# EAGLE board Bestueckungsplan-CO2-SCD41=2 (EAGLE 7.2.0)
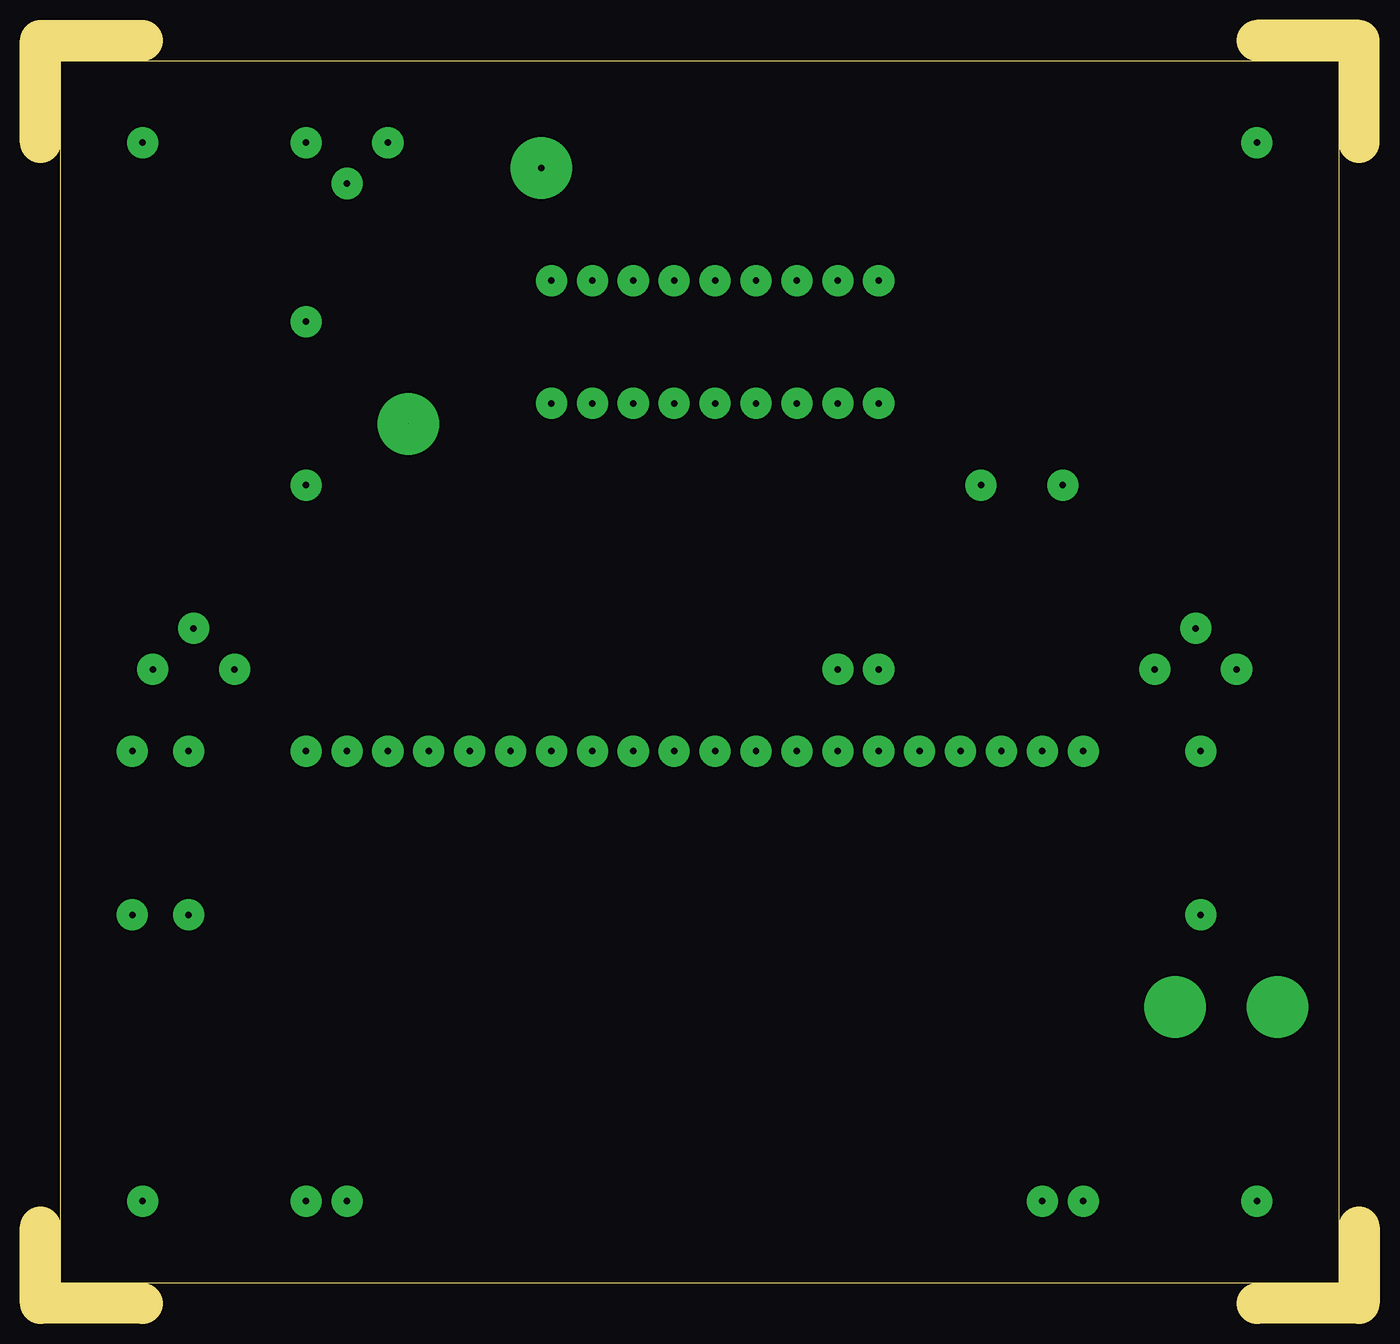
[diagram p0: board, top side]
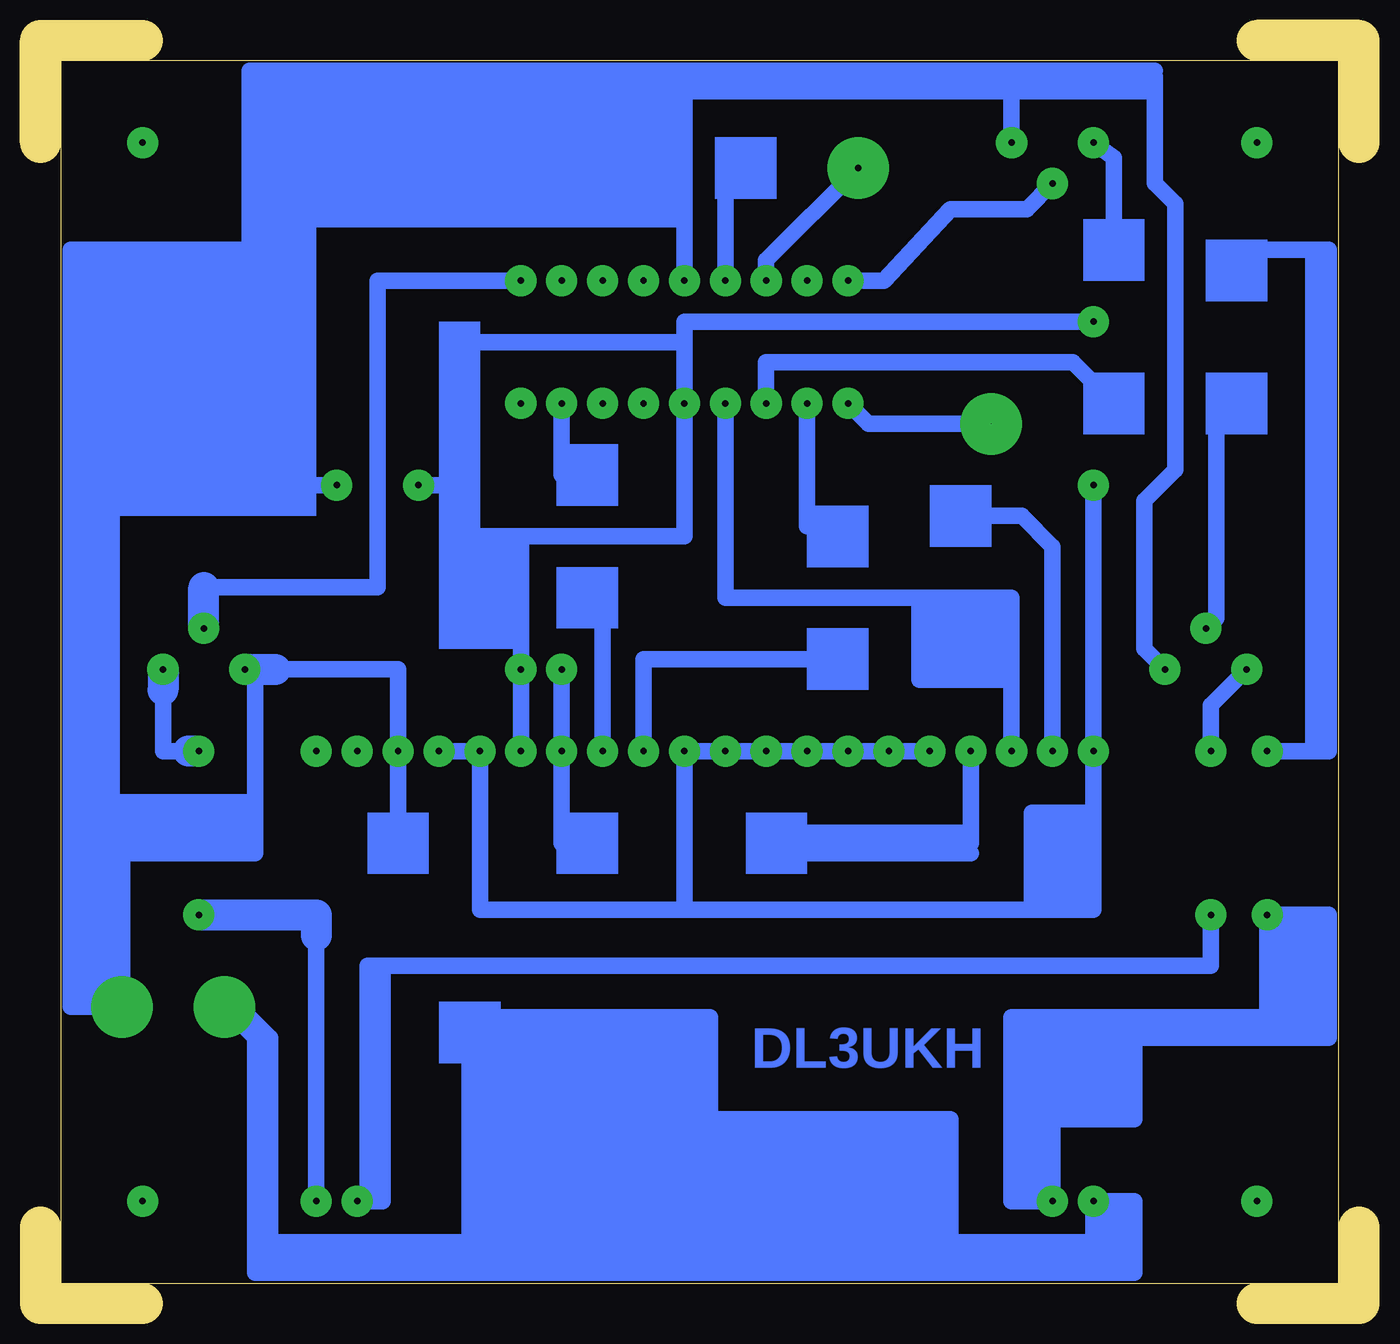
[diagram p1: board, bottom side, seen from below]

Size 81.91 x 78.42 mm. Coordinates in mm from the lower left corner, seen from the top.
Outline: 81.91,72.07 81.91,78.42 75.56,78.42
Outline: 81.91,4.76 81.91,0 75.56,0
Outline: 6.35,0 0,0 0,4.76
Outline: 0,72.07 0,78.42 6.35,78.42
Outline: 80.64,77.15 80.64,1.27 1.27,1.27 1.27,77.15 80.64,77.15
Copper layers (1*16): Top 0.035mm / dielectric 1.5mm / Bottom 0.035mm
Design rules "default": minimum track width 10mil, minimum drill 24mil, track to track 8mil, track to pad 8mil, pad to pad 8mil, via to via 8mil, smd to smd 8mil, copper to edge 40mil, drill to drill 8mil, minimum pad ring 10mil, minimum via ring 8mil, stop-mask expansion 4mil, vias tented up to drill 0mil, thermal gap 10mil

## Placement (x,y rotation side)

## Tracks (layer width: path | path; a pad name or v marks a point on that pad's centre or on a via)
S$1  (via drill 0.4 pad 1.93)
  Bottom 1.016: v58.42,50.8 55.88,50.8
S$2  (via drill 0.4 pad 1.93)
  other vias: 31.75,34.29
S$3  (via drill 0.4 pad 1.93)
  Bottom 1.016: v36.83,55.88 36.83,58.42 17.78,58.42 15.24,55.88
S$4  (via drill 0.4 pad 1.93)
  Bottom 1.016: v34.29,55.88 34.29,48.26 32.38,48.26
S$5  (via drill 0.4 pad 1.93)
  Bottom 1.016: v49.53,55.88 49.53,51.44 47.94,51.44
S$6  (via drill 0.4 pad 1.93)
  Bottom 1.016: v12.06,39.37 13.33,40.64 13.33,49.85 11.43,51.75 11.43,68.26 12.7,69.53 12.7,75.25 | 12.7,75.25 12.7,76.2 21.59,76.2 | 68.26,72.07 68.26,75.25 | 68.26,75.25 68.26,76.2 | 68.26,76.2 67.94,76.2 | 67.94,76.2 41.91,76.2 | 41.91,76.2 41.91,75.25 | 41.91,75.25 41.91,67.31 | 41.91,67.31 v41.91,63.5 | 41.91,76.2 33.97,76.2 | 33.97,76.2 21.59,76.2 | v21.59,72.07 21.59,76.2 | 33.97,76.2 20.95,75.25 | 68.26,76.2 68.26,76.52 | 68.26,76.52 67.94,76.52 | 67.94,76.52 12.7,76.52 | 41.91,75.25 68.26,75.25 | 41.91,75.25 20.95,75.25 | 12.7,75.25 20.95,75.25 | 67.94,76.2 67.94,76.52 | 68.26,76.52 68.9,76.52 68.9,64.14 | 41.91,67.31 68.58,67.31
S$7  (via drill 0.4 pad 1.93)
  other vias: 49.53,63.5
S$8  (via drill 0.4 pad 1.93)
  other vias: 6.35,6.35
S$9  (via drill 0.4 pad 1.93)
  other vias: 6.35,72.07
S$10  (via drill 0.01 pad 3.81, 0.4 pad 1.93)
  Bottom 1.016: v36.83,63.5 36.83,64.77 v31.11,70.48 | v31.75,55.88 30.48,54.61 v22.86,54.61 | v19.05,34.29 19.05,46.99 20.95,48.9 24.77,48.9
S$11  (via drill 0.4 pad 1.93)
  other vias: 34.29,34.29
S$12  (via drill 0.4 pad 1.93)
  Bottom 1.016: 60.64,20.95 60.33,20.95 9.21,20.95 v9.21,24.13 | 60.64,20.95 60.64,6.35 61.6,6.35 | 61.6,6.35 v62.23,6.35 | 61.6,6.35 61.6,20.95 60.64,20.95
S$13  (via drill 0.4 pad 1.93)
  other vias: 16.51,60.96
S$14  (via drill 0.4 pad 1.93)
  Bottom 1.016: v44.45,34.29 44.45,40.01 32.38,40.01
S$15  (via drill 0.4 pad 1.93)
  Bottom 1.016: v24.13,34.29 24.13,29.21 | 24.13,29.21 24.13,28.57 35.24,28.57 | 24.13,29.21 34.93,29.21
S$16  (via drill 0.4 pad 1.93)
  Bottom 1.016: v16.51,72.07 15.24,71.12 15.24,65.41
S$17  (via drill 0.4 pad 1.93)
  Bottom 1.016: v9.53,41.91 8.89,42.55 8.89,55.25
S$18  (via drill 0.4 pad 1.93)
  Bottom 1.016: 13.65,16.51 6.03,16.51 5.71,16.51 | 19.05,17.78 21.59,17.78 21.59,6.35 v19.05,6.35 19.05,11.43 | 19.05,17.78 13.97,17.78 | 13.97,17.78 5.71,17.78 | 5.71,17.78 v5.71,24.13 1.91,24.13 1.91,16.51 5.71,16.51 | 19.05,11.43 19.05,17.78 | 13.97,17.14 13.97,11.43 19.05,11.43 | 13.97,17.14 13.97,17.78 | 5.71,16.51 5.71,17.14 | 5.71,17.78 5.71,17.14 | 5.71,17.14 13.97,17.14
S$19  (via drill 0.4 pad 1.93)
  Bottom 1.016: v64.77,6.35 64.77,22.86
  Bottom 1.93: v72.07,24.13 64.77,24.13 64.77,22.86
S$20  (via drill 0.4 pad 1.93)
  Bottom 1.016: v63.5,50.8 67.63,50.8
S$21  (via drill 0.4 pad 1.93)
  other vias: 34.29,63.5
S$22  (via drill 0.4 pad 1.93)
  other vias: 52.07,55.88
S$23  (via drill 0.4 pad 1.93)
  Bottom 1.016: v16.51,50.8 v16.51,34.29 16.51,30.48 | 16.51,30.48 16.51,24.45 20.32,24.45 | 20.32,24.45 41.91,24.45 | v26.67,34.29 v29.21,34.29 v36.83,34.29 v41.91,34.29 41.91,24.45 | v57.15,34.29 v54.61,34.29 54.61,24.45 41.91,24.45 | 16.51,30.48 20.32,30.48 20.32,24.45
S$24  (via drill 0.4 pad 1.93)
  Bottom 1.016: v46.99,34.29 46.99,42.86
S$25  (via drill 0.4 pad 1.93)
  other vias: 62.23,34.29
S$26  (via drill 0.4 pad 1.93)
  other vias: 64.77,34.29
S$27  (via drill 0.4 pad 1.93)
  Bottom 1.016: v5.71,34.29 3.49,34.29 2.86,34.29 | 2.86,34.29 2.86,65.41 | 2.86,65.41 8.89,65.41 | 2.86,65.41 1.91,65.41 1.91,34.29 2.86,34.29
S$28  (via drill 0.01 pad 3.81, 0.4 pad 1.93)
  Bottom 1.016: 54.93,17.78 40.32,17.78 40.32,11.43 | 16.51,3.81 v16.51,6.35 13.97,6.35 13.97,2.54 | 16.51,3.81 16.51,2.54 | 16.51,2.54 55.25,2.54 | 55.25,2.54 55.25,11.43 | 55.25,11.43 55.25,16.83 | 55.25,2.54 68.58,2.54 | 68.58,2.54 68.58,3.81 | 68.58,3.81 68.58,16.51 | 68.58,16.51 v70.48,18.41 | 13.97,2.54 16.51,2.54 | 16.51,3.81 68.58,3.81 | 13.97,2.54 13.97,1.91 68.58,1.91 68.58,2.54 | 25.4,3.17 25.4,11.43 40.32,11.43 | 40.32,11.43 55.25,11.43 | 68.58,16.51 67.63,16.51 | 67.63,16.51 67.63,3.17 | 67.63,16.51 70.17,19.05
S$29  (via drill 0.4 pad 1.93)
  other vias: 75.56,6.35
S$30  (via drill 0.4 pad 1.93)
  Bottom 1.016: v52.07,63.5 60.96,63.5 60.96,44.45 62.23,44.45 63.82,44.45 71.75,44.45
  Bottom 1.93: v71.75,41.91 71.75,44.45
S$31  (via drill 0.4 pad 1.93)
  Bottom 1.016: v31.75,63.5 29.53,63.5 25.4,67.94 20.64,67.94 v19.05,69.53
S$32  (via drill 0.01 pad 3.81, 0.4 pad 1.93)
  Bottom 1.016: 68.26,65.41 68.26,62.23 77.47,62.23 | 68.26,65.41 77.47,65.41 | 77.47,65.41 80.01,65.41 80.01,31.11 | 77.47,65.41 77.47,62.23 | 80.01,31.11 80.01,18.41 v76.83,18.41 76.83,31.11 | 77.47,62.23 77.47,31.11 | 77.47,31.11 80.01,31.11 | 77.15,27.94 68.58,27.94 68.58,31.11 | 77.47,31.11 76.83,31.11 | 76.83,31.11 68.58,31.11 | 68.58,31.11 68.58,38.74 v69.21,39.37 | 67.31,39.37 59.69,39.37 v59.69,34.29 59.69,28.89 | 68.26,65.41 68.26,67.63
  Bottom 1.93: v69.21,39.37 67.31,39.37
S$33  (via drill 0.4 pad 1.93)
  Bottom 1.016: 72.71,34.29 74.3,34.29 74.3,38.1
  Bottom 1.93: v74.3,39.37 74.3,38.1 | v72.07,34.29 72.71,34.29
S$34  (via drill 0.4 pad 1.93)
  other vias: 75.56,72.07
S$35  (via drill 0.4 pad 1.93)
  Bottom 1.016: v49.53,39.37 v49.53,34.29 49.53,28.57
S$36
  Bottom 1.016: 24.13,27.94 34.29,27.94
S$37  (via drill 0.4 pad 1.93)
  other vias: 44.45,55.88
S$38  (via drill 0.4 pad 1.93)
  other vias: 46.99,63.5
S$39  (via drill 0.4 pad 1.93)
  Bottom 1.016: v39.37,63.5 39.37,69.21 37.78,69.21 37.78,70.8
S$40  (via drill 0.01 pad 3.81)
  other vias: 90.49,41.91 31.11,70.48 22.86,54.61 70.48,18.41 76.83,18.41
S$41  (via drill 0.4 pad 1.93)
  other vias: 44.45,63.5
S$42  (via drill 0.4 pad 1.93)
  Bottom 1.016: v6.98,39.37 9.21,37.15 v9.21,34.29
S$43
  Bottom 1.016: 67.63,72.07 67.63,75.56
S$44  (via drill 0.4 pad 1.93)
  Bottom 1.016: v21.59,34.29 21.59,38.74 | 21.59,38.74 21.59,43.82 27.3,43.82 | 27.3,43.82 39.37,43.82 v39.37,55.88 | 21.59,38.74 27.3,38.74 27.3,43.82
S$45  (via drill 0.4 pad 1.93)
  other vias: 46.99,55.88
S$46  (via drill 0.4 pad 1.93)
  Bottom 1.016: 52.07,47.62 41.91,47.62 v41.91,55.88 41.91,59.69 | 52.07,47.62 55.25,47.62 52.07,42.55 | v52.07,34.29 v52.07,39.37 52.07,42.55 | 41.91,59.69 41.91,60.96 16.51,60.96 | 52.07,42.55 55.25,42.55 | 56.52,59.69 41.91,59.69 | 52.07,42.55 52.07,47.62
S$48  (via drill 0.4 pad 1.93)
  other vias: 39.37,34.29
(copper drawn outside any net)
  shapes: Bottom area x36

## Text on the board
Bottom: DL3UKH
Pads: AUF BESTÜCKUNGS-SEITE GESEHEN
Vias: 1 | 2 | 1 | 2 | +5V | - | +5V | -
tOrigins: PIC16F1827 | 2N7000 | 1 | Links oben ist | immer PIN 1 | D | S | D | Br. | BOHRUNGEN: | G | alles 0.8mm | 1 | 4Stck. Befestigungsbohr... 3,5mm | Br. | 10K | Leiterplatte: | Br. | 1,5mm dick | 47n | Cevausit | Br. | Br. | Für Anschlüsse | D | D | Siehe Stromlaufplan | 47n | Auf Leiterzugseite anlöten | 680 | 680 | 680 | 40 | 35 | 30 | 25 | 21 | Br. | Br. | Für die 8stck. Brücken | Br. | Br. | Die Lötinseln | Vergleiche mit Stromlaufplan | 19 | Auf Leiterzugseite anlöten | 2 | 1 | LCD-Display | 20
